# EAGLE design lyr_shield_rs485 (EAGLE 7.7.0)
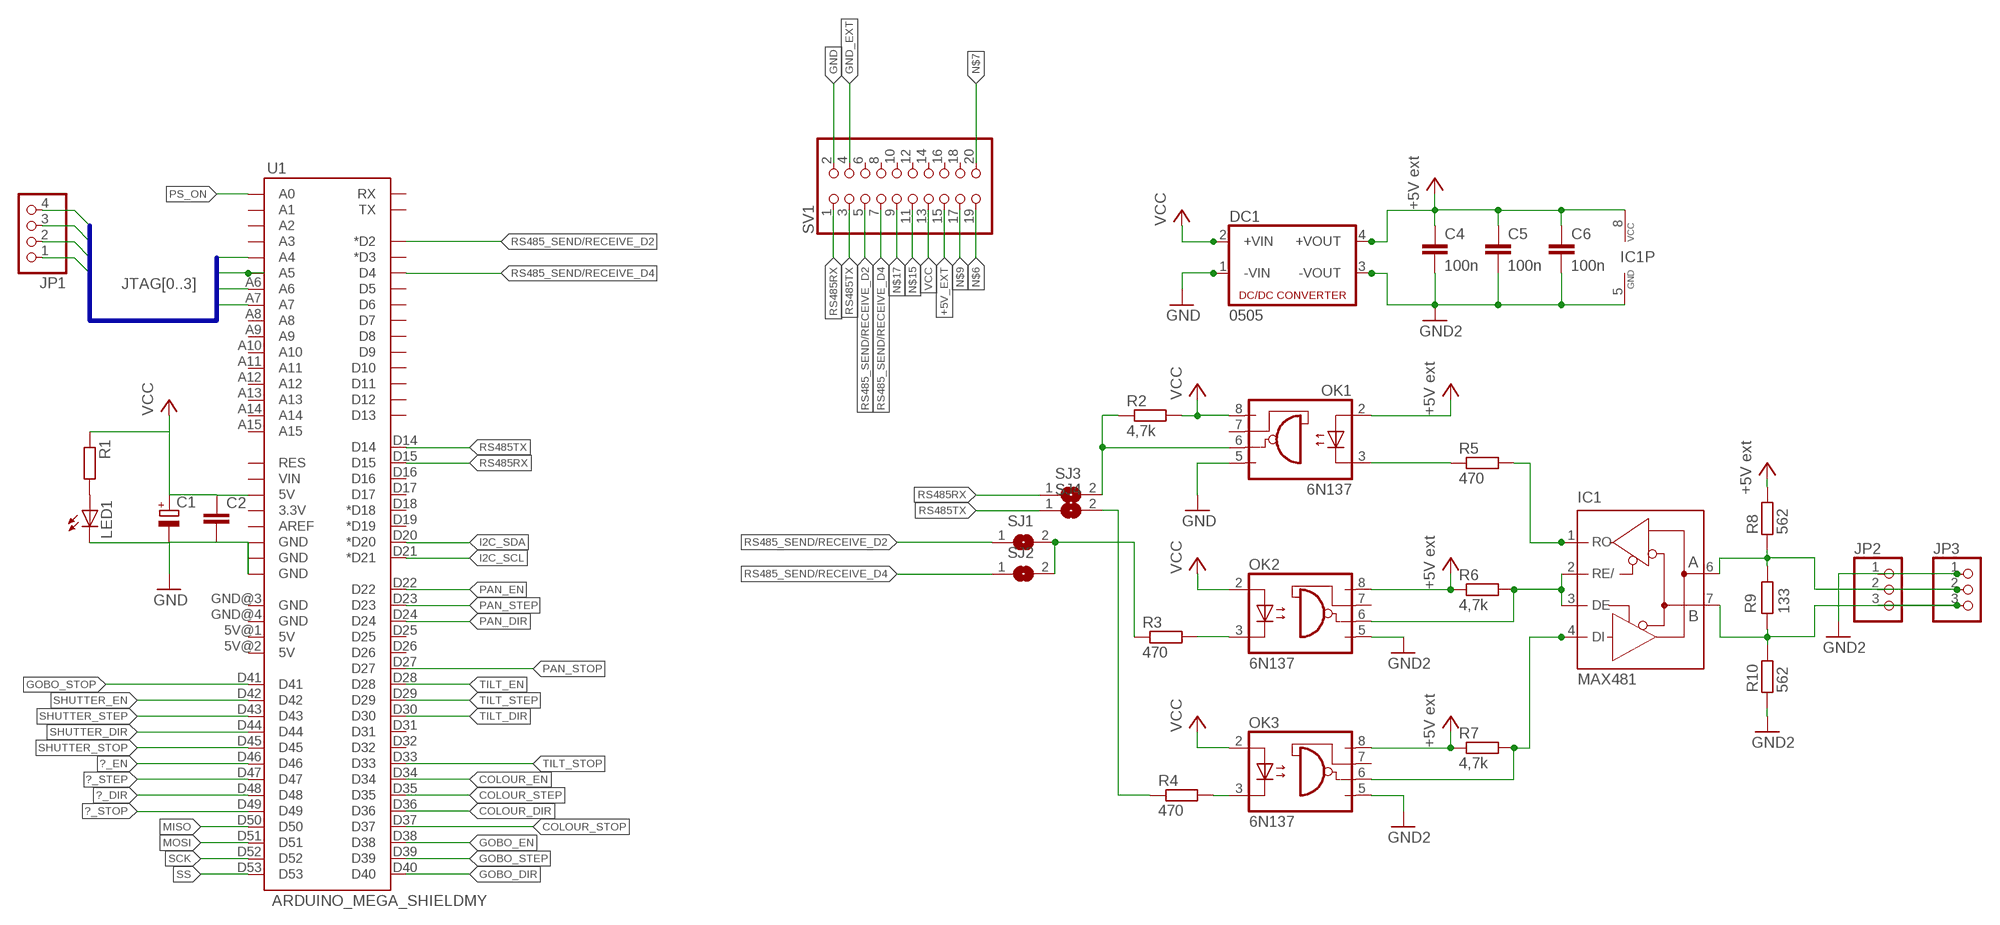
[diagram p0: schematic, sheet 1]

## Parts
C1  CPOL-EUE5-8.5  [E5-8,5]
C2  C-EU025-025X050  [C025-025X050]
C4  100n  C7.5/3  [C7.5B3]
C5  100n  C7.5/3  [C7.5B3]
C6  100n  C7.5/3  [C7.5B3]
DC1  0505  NME  [NME]
IC1  MAX481  MAX481CPA  [DIL08]
JP1  PINHD-1X4  [1X04]
JP2  + - 0  PINHD-1X3  [1X03]
JP3  + - 0  PINHD-1X3  [1X03]
LED1  LED5MM  [LED5MM]
OK1  6N137  [DIL08]
OK2  6N137  [DIL08]
OK3  6N137  [DIL08]
R1  R-EU_0207/10  [0207/10]
R2  4,7k  R-EU_0207/10  [0207/10]
R3  470  R-EU_0207/10  [0207/10]
R4  470  R-EU_0207/10  [0207/10]
R5  470  R-EU_0207/10  [0207/10]
R6  4,7k  R-EU_0207/10  [0207/10]
R7  4,7k  R-EU_0207/10  [0207/10]
R8  562  R-EU_0207/10  [0207/10]
R9  133  R-EU_0207/10  [0207/10]
R10  562  R-EU_0207/10  [0207/10]
SJ1  SJ  [SJ]
SJ2  SJ  [SJ]
SJ3  SJ  [SJ]
SJ4  SJ  [SJ]
SV1  PINHD-2X10/90  [2X10/90]
U1  ARDUINO_MEGA_SHIELDMY  [MY_ARDUINO_MEGA_SHIELD]

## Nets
+5V [SUPPLY]: OK3.8(VCC) R7.1 ; supply symbol labelled +5V ext
+5V_EXT [SUPPLY]: C4.1 C5.1 C6.1 DC1.4(+VOUT) IC1.8(VCC) OK1.2(A) OK2.8(VCC) R6.1 R8.2 SV1.15 ; supply symbol labelled +5V ext
?_DIR: U1.D48
?_EN: U1.D46
?_STEP: U1.D47
?_STOP: U1.D49
COLOUR_EN: U1.D34
COLOUR_STEP: U1.D35
COLOUR_STOP: U1.D37
D2: R4.1 SJ4.2
GND [SUPPLY]: C1.- C2.2 DC1.1(-VIN) LED1.K(C) OK1.5(GND) SV1.2 U1.GND@0(GND) U1.GND@1(GND) U1.GND@2(GND)
GND_EXT [SUPPLY]: C4.2 C5.2 C6.2 DC1.3(-VOUT) IC1.5(GND) JP2.1 JP3.1 OK2.5(GND) OK3.5(GND) R10.1 SV1.4 ; supply symbol labelled GND2
GOBO_DIR: U1.D40
GOBO_EN: U1.D38
GOBO_STEP: U1.D39
GOBO_STOP: U1.D41
I2C_SCL: U1.D21(*D21)
I2C_SDA: U1.D20(*D20)
JTAG0: JP1.1 U1.A4
JTAG1: JP1.2 U1.A5
JTAG2: JP1.3 U1.A6
JTAG3: JP1.4 U1.A7
MISO: U1.D50
MOSI: U1.D51
N$1: R3.1 SJ1.2 SJ2.2
N$3: OK2.3(C) R3.2
N$5: OK3.3(C) R4.2
N$6: IC1.2(RE/) IC1.3(DE) OK2.6(VO) R6.2 SV1.19
N$7: IC1.4(DI) OK3.6(VO) R7.2 SV1.20
N$8: OK1.3(C) R5.1
N$9: IC1.1(RO) R5.2 SV1.17
N$10: OK1.6(VO) R2.1 SJ3.2
N$15: IC1.7(B) JP2.3 JP3.3 R9.2 R10.2 SV1.11
N$17: IC1.6(A) JP2.2 JP3.2 R8.1 R9.1 SV1.9
N$55: LED1.A R1.2
PAN_DIR: U1.D24
PAN_EN: U1.D22
PAN_STEP: U1.D23
PAN_STOP: U1.D27
PS_ON: U1.A0
RS485_SEND/RECEIVE_D2: SJ1.1 SV1.5 U1.D2(*D2)
RS485_SEND/RECEIVE_D4: SJ2.1 SV1.7 U1.D4
RS485RX: SJ3.1 SV1.1 U1.D15
RS485TX: SJ4.1 SV1.3 U1.D14
SCK: U1.D52
SHUTTER_DIR: U1.D44
SHUTTER_EN: U1.D42
SHUTTER_STEP: U1.D43
SHUTTER_STOP: U1.D45
SS: U1.D53
TILT_DIR: U1.D30
TILT_EN: U1.D28
TILT_STEP: U1.D29
TILT_STOP: U1.D33
VCC [SUPPLY]: C1.+ C2.1 DC1.2(+VIN) OK1.8(VCC) OK2.2(A) OK3.2(A) R1.1 R2.2 SV1.13 U1.5V@0(5V)
Unconnected: OK1.7(VE) OK2.7(VE) OK3.7(VE) SV1.6 SV1.8 SV1.10 SV1.12 SV1.14 SV1.16 SV1.18 U1.3.3V U1.5V@1(5V) U1.5V@2(5V) U1.A1 U1.A2 U1.A3 U1.A8 U1.A9 U1.A10 U1.A11 U1.A12 U1.A13 U1.A14 U1.A15 U1.AREF U1.D3(*D3) U1.D5 U1.D6 U1.D7 U1.D8 U1.D9 U1.D10 U1.D11 U1.D12 U1.D13 U1.D16 U1.D17 U1.D18(*D18) U1.D19(*D19) U1.D25 U1.D26 U1.D31 U1.D32 U1.D36 U1.GND@3(GND) U1.GND@4(GND) U1.RES U1.RX U1.TX U1.VIN

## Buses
JTAG[0..3]

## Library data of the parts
C1 = rcl:CPOL-EU: POLARIZED CAPACITOR, European symbol
C2 = rcl:C-EU: CAPACITOR, European symbol
C4-C6 = capacitor-wima:C: CAPACITOR
DC1 = dc-dc-converter:NME: DC-DC CONVERTER; MF: C & D TECHNOLOGIES, INC; MPN: NME1205D; OC_FARNELL: 1021466; OC_NEWARK: 98B8198
IC1 = mathertel:MAX481CPA: RS485 TRANSEIVER; MPN: MAX481CPA+; OC_FARNELL: unknown; OC_NEWARK: 99K3445
JP1 = pinhead:PINHD-1X4: PIN HEADER
JP2 JP3 = mathertel:PINHD-1X3: PIN HEADER
LED1 = RepRapjr:LED: LED
OK1-OK3 = optocoupler:6N137: MOTOROLA OPTO COUPLER; MPN: 6N137; OC_FARNELL: 1328376; OC_NEWARK: 52M1895
R1 = rcl:R-EU_: RESISTOR, European symbol
R2-R10 = resistor:R-EU_: RESISTOR, European symbol
SJ1-SJ4 = jumper:SJ: SMD solder JUMPER
SV1 = pinhead:PINHD-2X10: PIN HEADER
U1 = RepRapjr:ARDUINO_MEGA_SHIELD

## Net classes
0 default: width 0.406 mm
1 SUPPLY: width 0.813 mm
2 gnd: width 0.813 mm

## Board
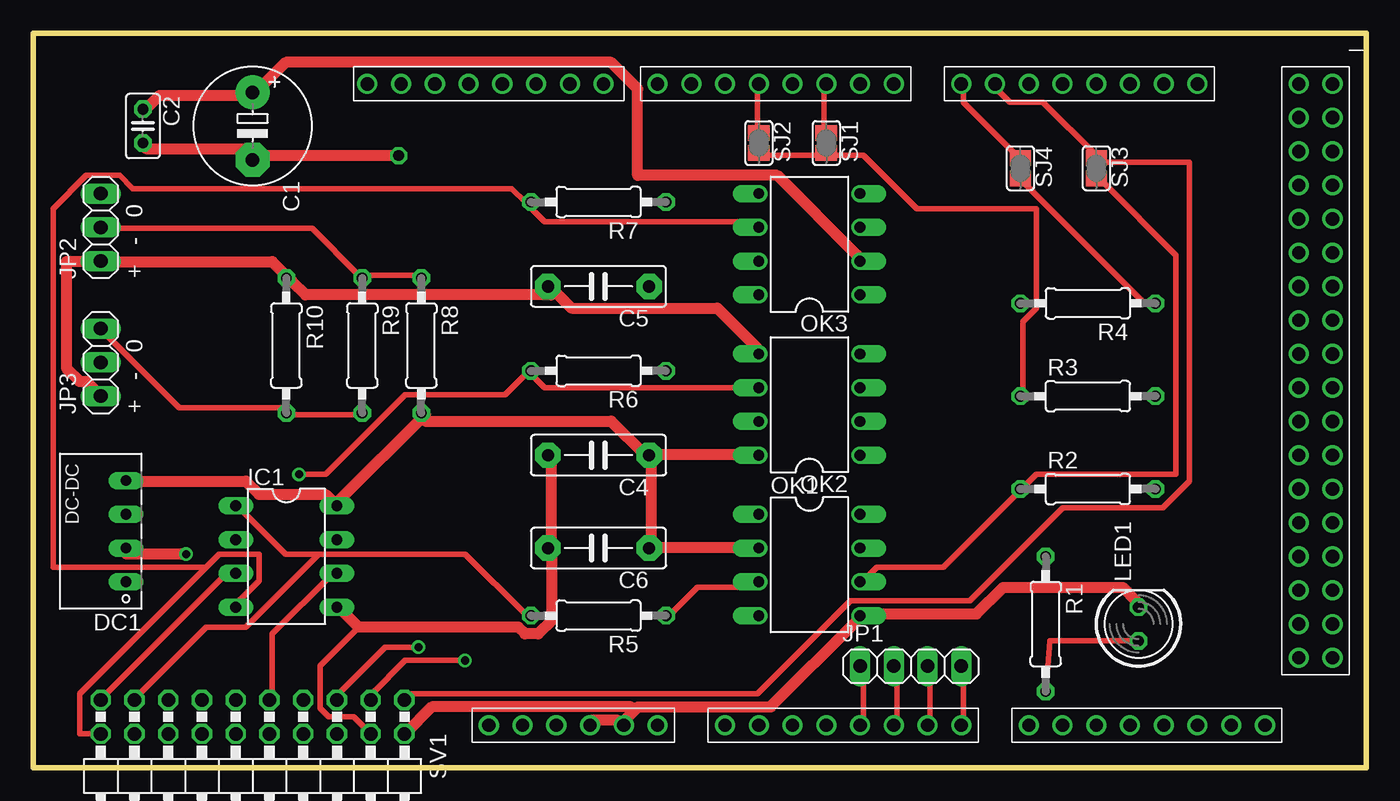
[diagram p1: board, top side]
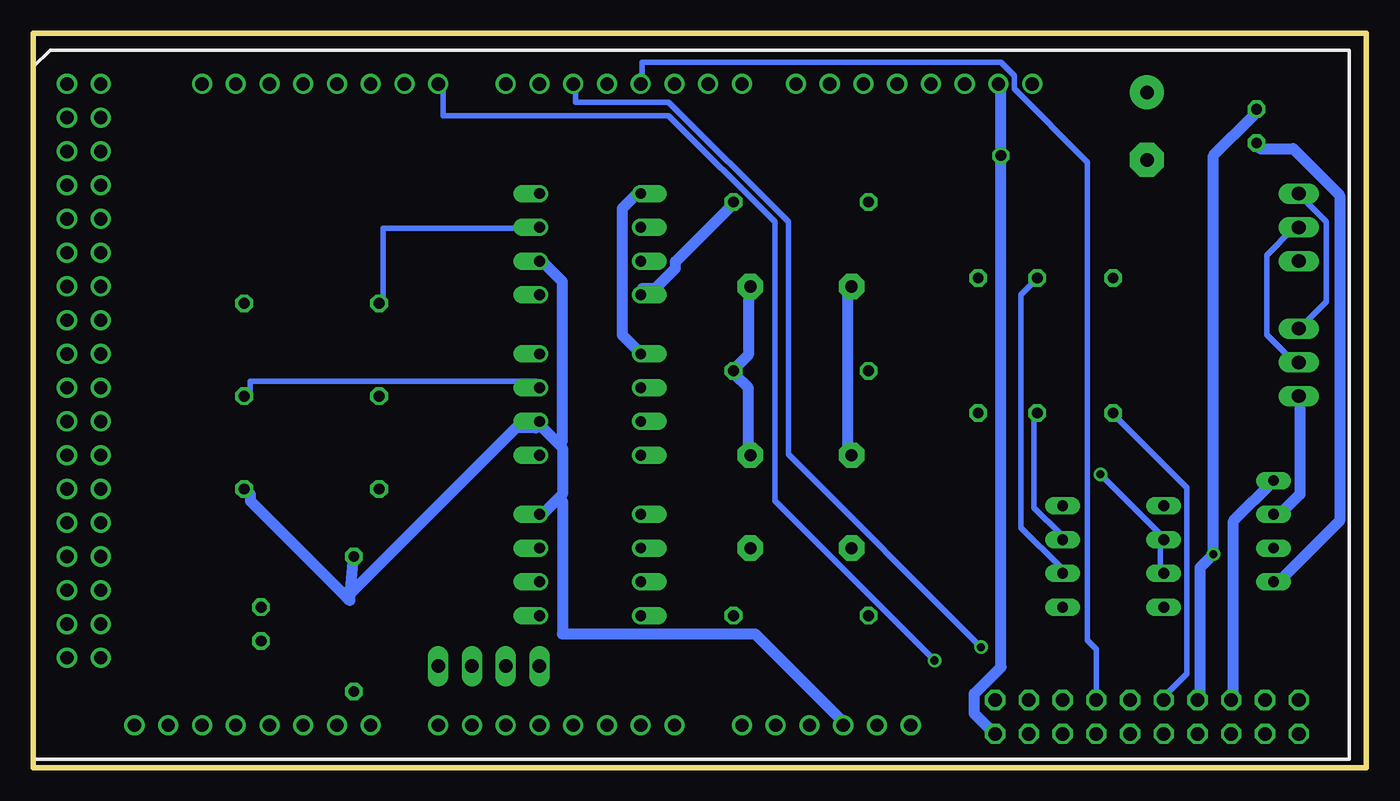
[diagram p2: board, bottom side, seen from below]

Size 100.33 x 55.24 mm. Coordinates in mm from the lower left corner, seen from the top.
Outline: 100.33,0 100.33,55.24 0,55.24 0,0 100.33,0
Copper layers (1*16): Top 0.035mm / dielectric 1.5mm / Bottom 0.035mm
Design rules "default": minimum track width 10mil, minimum drill 24mil, track to track 8mil, track to pad 8mil, pad to pad 8mil, via to via 8mil, smd to smd 8mil, copper to edge 40mil, drill to drill 8mil, minimum pad ring 10mil, minimum via ring 8mil, stop-mask expansion 4mil, vias tented up to drill 0mil, thermal gap 10mil

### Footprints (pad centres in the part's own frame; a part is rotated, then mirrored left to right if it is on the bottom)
E5-8,5 = drill 1.016 pad 2.54: + -2.54,0 | drill 1.016 pad 2.54 octagon: - 2.54,0
C025-025X050 = drill 0.813 octagon: 1 -1.27,0; 2 1.27,0
C7.5B3 = drill 0.914 pad 1.905 octagon: 1 -3.81,0; 2 3.81,0
NME = drill 0.813 long: 1 0,3.81; 2 0,1.27; 3 0,-1.27; 4 0,-3.81
DIL08 = drill 0.813 long: 1 -3.81,-3.81; 2 -1.27,-3.81; 3 1.27,-3.81; 4 3.81,-3.81; 5 3.81,3.81; 6 1.27,3.81; 7 -1.27,3.81; 8 -3.81,3.81
1X04 = drill 1.016 long: 1 -3.81,0; 2 -1.27,0; 3 1.27,0; 4 3.81,0
1X03 = drill 1.016 long: 1 -2.54,0; 2 0,0; 3 2.54,0
LED5MM = drill 0.813 octagon: A -1.27,0; K 1.27,0
DIL08' = drill 0.813 offset: 1 -3.81,-3.81; 2 -1.27,-3.81; 3 1.27,-3.81; 4 3.81,-3.81; 5 3.81,3.81; 6 1.27,3.81; 7 -1.27,3.81; 8 -3.81,3.81
0207/10 = drill 0.813 octagon: 1 -5.08,0; 2 5.08,0
SJ = smd 1.168 x 1.6: 1 -0.762,0; 2 0.762,0
2X10/90 = drill 1.016 octagon: 1 -11.43,-6.35; 2 -11.43,-3.81; 3 -8.89,-6.35; 4 -8.89,-3.81; 5 -6.35,-6.35; 6 -6.35,-3.81; 7 -3.81,-6.35; 8 -3.81,-3.81; 9 -1.27,-6.35; 10 -1.27,-3.81; 11 1.27,-6.35; 12 1.27,-3.81; 13 3.81,-6.35; 14 3.81,-3.81; 15 6.35,-6.35; 16 6.35,-3.81; 17 8.89,-6.35; 18 8.89,-3.81; 19 11.43,-6.35; 20 11.43,-3.81
MY_ARDUINO_MEGA_SHIELD = drill 1 pad 1.422: 3.3V 63.5,50.8; 5V@0 60.96,50.8; 5V@1 5.08,2.54; 5V@2 2.54,2.54; A0 48.26,50.8; A1 45.72,50.8; A2 43.18,50.8; A3 40.64,50.8; A4 38.1,50.8; A5 35.56,50.8; A6 33.02,50.8; A7 30.48,50.8; A8 25.4,50.8; A9 22.86,50.8; A10 20.32,50.8; A11 17.78,50.8; A12 15.24,50.8; A13 12.7,50.8; A14 10.16,50.8; A15 7.62,50.8; AREF 75.184,2.54; D2 40.64,2.54; D3 43.18,2.54; D4 45.72,2.54; D5 48.26,2.54; D6 50.8,2.54; D7 53.34,2.54; D8 57.404,2.54; D9 59.944,2.54; D10 62.484,2.54; D11 65.024,2.54; D12 67.564,2.54; D13 70.104,2.54; D14 30.48,2.54; D15 27.94,2.54; D16 25.4,2.54; D17 22.86,2.54; D18 20.32,2.54; D19 17.78,2.54; D20 15.24,2.54; D21 12.7,2.54; D22 5.08,5.08; D23 2.54,5.08; D24 5.08,7.62; D25 2.54,7.62; D26 5.08,10.16; D27 2.54,10.16; D28 5.08,12.7; D29 2.54,12.7; D30 5.08,15.24; D31 2.54,15.24; D32 5.08,17.78; D33 2.54,17.78; D34 5.08,20.32; D35 2.54,20.32; D36 5.08,22.86; D37 2.54,22.86; D38 5.08,25.4; D39 2.54,25.4; D40 5.08,27.94; D41 2.54,27.94; D42 5.08,30.48; D43 2.54,30.48; D44 5.08,33.02; D45 2.54,33.02; D46 5.08,35.56; D47 2.54,35.56; D48 5.08,38.1; D49 2.54,38.1; D50 5.08,40.64; D51 2.54,40.64; D52 5.08,43.18; D53 2.54,43.18; GND@0 58.42,50.8; GND@1 55.88,50.8; GND@2 72.644,2.54; GND@3 5.08,45.72; GND@4 2.54,45.72; RES 66.04,50.8; RX 35.56,2.54; TX 38.1,2.54; VIN 53.34,50.8

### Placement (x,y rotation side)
C1  16.51,48.26 270 top
C2  8.26,48.26 270 top
C4  42.55,23.5 180 top
C5  42.55,36.2 180 top
C6  42.55,16.51 180 top
DC1  6.99,17.78 180 top
IC1  19.05,15.88 270 top
JP1  66.04,7.62 0 top
JP2  5.08,40.64 90 top
JP3  5.08,30.48 90 top
LED1  83.19,10.79 90 top
OK1  6N137  [DIL08']  58.42,15.24 270 top
OK2  6N137  [DIL08']  58.42,27.3 90 top
OK3  6N137  [DIL08']  58.42,39.37 90 top
R1  76.2,10.79 270 top
R2  79.38,20.95 0 top
R3  79.38,27.94 0 top
R4  79.38,34.92 180 top
R5  42.55,11.43 180 top
R6  42.55,29.84 180 top
R7  42.55,42.55 180 top
R8  29.21,31.75 270 top
R9  24.77,31.75 270 top
R10  19.05,31.75 270 top
SJ1  59.69,46.99 270 top
SJ2  54.61,46.99 270 top
SJ3  80.01,45.09 270 top
SJ4  74.3,45.09 270 top
SV1  16.51,-1.27 180 top
U1  100.33,53.98 180 top

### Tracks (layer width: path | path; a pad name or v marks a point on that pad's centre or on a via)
+5V
  Bottom 0.813: R7.1 48,42.05 52,38.05 52,37.55 53.5,36.05 54.5,36.05 OK3.8
+5V_EXT
  Top 0.813: 46.5,16.55 54.5,16.55 OK1.2 | OK2.8 54.5,23.55 46.5,23.55 C4.1 | 46.5,16.55 46.5,23.05 C4.1 | 46.5,16.55 C6.1 | DC1.4 7,21.55 16,21.55 17,20.55 22,20.55 22.5,20.05 IC1.8 23,20.05 29.5,26.55 R8.2 29.5,26.05 43.5,26.05 46,23.55 C4.1
  Bottom 0.813: C5.1 46.5,36.05 46.5,31.05 47.5,30.05 R6.1 47.5,29.55 46.5,28.55 46.5,23.55 C4.1 | DC1.4 7,21.55 10,18.55 10,5.55 SV1.15
D2
  Top 0.406: SJ4.2 74.5,44.05 83.5,35.05 84,35.05 R4.1
GND  (via drill 0.8 pad 1.27)
  Top 0.813: C2.2 8.5,46.55 16,46.55 16.5,46.05 C1.- 17,46.05 27.48,46.05 v27.5,46.04 | 45.25,4.3 44.5,3.55 U1.GND@1 44,3.55 42,3.55 U1.GND@0 | 45.25,4.3 45.5,4.55 55.5,4.55 62,11.05 OK1.5 62.5,11.55 71,11.55 73,13.55 82,13.55 83,12.55 LED1.K | SV1.2 28,2.55 30,4.55 45,4.55 45.25,4.3
  Bottom 0.813: DC1.1 6.5,14.05 2,18.55 2,43.05 5.5,46.55 8,46.55 C2.2 | v27.5,46.04 27.5,7.55 29.5,5.55 29.5,4.05 28,2.55 SV1.2 | v27.5,46.04 27.5,51.05 U1.GND@2 27.5,51.25 v27.5,46.04
GND_EXT
  Top 0.406: 24.5,10.55 21.59,7.64 21.59,4.45 22.23,3.81 24.13,3.81 SV1.4
  Top 0.813: JP3.1 5,28.05 4,29.05 3.5,29.05 2.5,30.05 2.5,38.05 5,38.05 JP2.1 5.5,38.05 18,38.05 19,37.05 R10.1 19.5,36.55 20.5,35.55 39,35.55 C5.2 39,36.05 40.5,34.55 51.5,34.55 54.5,31.55 OK2.5 | IC1.5 23,12.05 24.5,10.55 36.5,10.55 37,10.05 38,10.05 39,11.05 39,16.05 C6.2 39,16.55 39,23.05 C4.2
  Bottom 0.813: DC1.3 6.5,19.05 5,20.55 5,27.55 JP3.1 | OK2.5 55,31.55 56,32.55 56,42.05 55,43.05 OK3.5 | C5.2 39,36.05 39,23.55 C4.2
JTAG0
  Top 0.406: U1.A4 62.5,3.55 62.5,7.55 JP1.1
JTAG1
  Top 0.406: U1.A5 65,3.55 65,7.55 JP1.2
JTAG2
  Top 0.406: U1.A6 67.5,3.55 67.5,7.55 JP1.3
JTAG3
  Top 0.406: U1.A7 70,3.55 70,7.55 JP1.4
N$1
  Top 0.406: SJ2.2 55,46.05 59.5,46.05 SJ1.2 60,46.05 62.5,46.05 66.5,42.05 75.5,42.05 75.5,34.55 74.5,33.55 74.5,28.05 R3.1
N$3
  Bottom 0.406: OK2.3 62.5,29.05 84,29.05 84,28.05 R3.2
N$5
  Bottom 0.406: OK3.3 62.5,40.55 74,40.55 74,35.05 R4.2
N$6  (via drill 0.61)
  Top 0.406: OK2.6 54.5,28.55 38.5,28.55 37.5,29.55 R6.2 37,29.55 35.5,28.05 28,28.05 22,22.05 v20,22.05 | SV1.19 5.5,5.55 14.5,14.55 15,14.55 IC1.3
  Bottom 0.406: IC1.3 15.5,15.05 15.5,17.05 IC1.2 15.5,17.55 v20,22.05
N$7
  Top 0.406: OK3.6 54.5,41.05 38.5,41.05 37.5,42.05 R7.2 37,42.55 36,43.55 7.5,43.55 6.5,44.55 4,44.55 1.5,42.05 1.5,15.05 13,15.05 | 13,15.05 3.5,5.55 3.5,2.55 5,2.55 SV1.20 | 13,15.05 14,16.05 17,16.05 17,14.05 15.5,12.55 IC1.4
N$8
  Top 0.406: R5.1 48,11.55 50,13.55 54.5,13.55 OK1.3
N$9
  Top 0.406: 21.5,16.05 32.5,16.05 37,11.55 R5.2 | 21.5,16.05 19,16.05 15.5,19.55 IC1.1 | 21.5,16.05 16,10.55 13,10.55 8,5.55 SV1.17
N$10
  Top 0.406: SJ3.2 80.5,44.05 86,38.55 86,22.05 75.5,22.05 74.5,21.05 R2.1 74,20.55 68.5,15.05 63.5,15.05 62.5,14.05 OK1.6
N$15
  Top 0.406: R9.2 24.5,26.55 19.5,26.55 R10.2 19,27.05 11,27.05 5.5,32.55 JP3.3
  Bottom 0.406: IC1.7 23,17.55 25,19.55 25,26.55 R9.2 | SV1.11 15,5.55 13.5,7.05 13.5,21.05 19,26.55 R10.2 | JP2.3 5,43.05 3,41.05 3,35.05 5,33.05 JP3.3
N$17
  Top 0.406: IC1.6 22.5,14.55 18,10.05 18,5.55 SV1.9 | R8.1 29,37.05 25,37.05 R9.1 24.5,37.05 21,40.55 5.5,40.55 JP2.2
  Bottom 0.406: JP3.2 5.5,30.55 7.5,32.55 7.5,38.55 5.5,40.55 JP2.2 | IC1.6 23,15.05 26,18.05 26,35.55 25,36.55 R9.1
N$55
  Top 0.406: R1.2 76.5,9.55 83,9.55 LED1.A
RS485_SEND/RECEIVE_D2  (via drill 0.61)
  Top 0.406: SJ1.1 59.5,48.05 59.5,51.05 U1.D2 | v29,9.05 26.5,9.05 23,5.55 SV1.5
  Bottom 0.406: v29,9.05 43.5,23.55 43.5,41.05 52.5,50.05 59.5,50.05 59.5,51.05 U1.D2
RS485_SEND/RECEIVE_D4
  Top 0.406: SJ2.1 54.5,48.05 54.5,51.05 U1.D4
  Bottom 0.406: U1.D4 54.5,51.55 54.5,53.05 27.5,53.05 26.5,52.05 26.5,51.05 21,45.55 21,9.57 20.32,8.89 SV1.7
RS485RX
  Top 0.406: U1.D15 72.5,51.05 73.5,50.05 76,50.05 80,46.05 SJ3.1 80.5,45.55 87,45.55 87,21.55 85,19.55 77.5,19.55 70.5,12.55 61.5,12.55 54.5,5.55 28,5.55 SV1.1
RS485TX  (via drill 0.61)
  Top 0.406: SJ4.1 74,46.05 70,50.05 70,51.05 U1.D14 | v32.5,8.05 28,8.05 25.5,5.55 SV1.3
  Bottom 0.406: v32.5,8.05 44.5,20.05 44.5,41.05 52.5,49.05 69.5,49.05 69.5,51.05 U1.D14
VCC  (via drill 0.61)
  Top 0.813: C2.1 8.5,49.55 9.5,50.55 16.5,50.55 C1.+ 17,51.05 19,53.05 43.5,53.05 45.5,51.05 45.5,44.55 56,44.55 62,38.55 OK3.2 | v11.5,16.05 7,16.05 DC1.2
  Bottom 0.813: SV1.13 12.5,5.55 12.5,15.05 v11.5,16.05 11.5,46.05 8.5,49.05 C2.1 | 76.75,12.8 84,20.05 84,20.55 R2.2 | 76.75,12.8 76.5,12.55 R1.1 | 60.75,20.3 60.5,20.55 60.5,24.05 60.75,24.3 | 60.75,20.3 62,19.05 OK1.8 | 60.75,24.3 62,25.55 OK2.2 62.5,25.55 64,25.55 76.75,12.8 | OK3.2 62,38.05 60.5,36.55 60.5,24.55 60.75,24.3 | U1.5V@0 39.5,3.55 46,10.05 60.5,10.05 60.5,20.05 60.75,20.3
